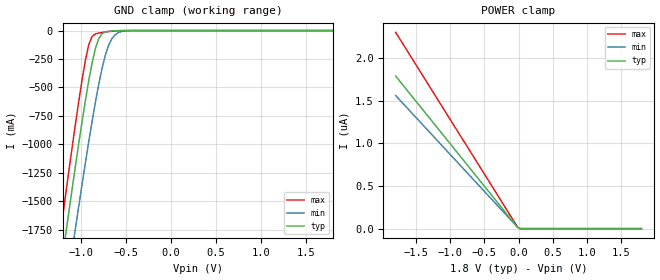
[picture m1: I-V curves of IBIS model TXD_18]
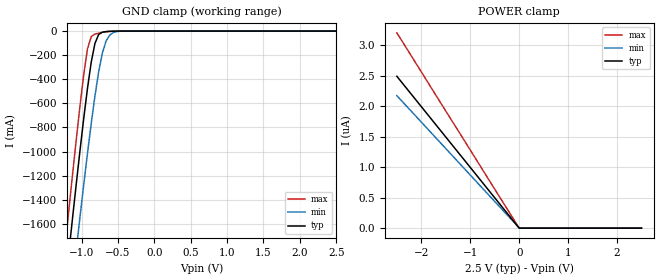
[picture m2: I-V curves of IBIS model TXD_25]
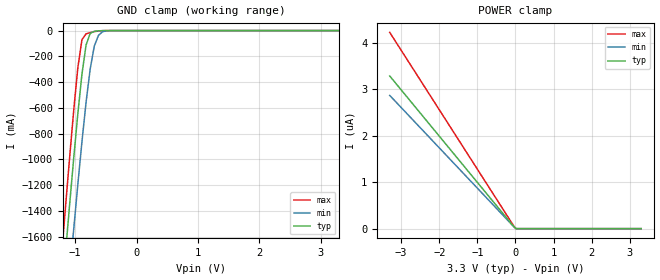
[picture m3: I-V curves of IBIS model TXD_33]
| IBIS file created by Layout Workbench Version 22.1.4.12161.401368   004
| Cadence Design Systems, Inc. 2011
[IBIS ver]   4.2
[File name]  iso6041.ibs
[File Rev]   1.5
[Date]   07 23, 2025
[Source]   Model built from TISPICED simulations at:
   Texas Instruments Incorporated.
   Analog-eLab, HPA 12500 TI Blvd
   Dallas, TX -75243
   For Support e-mail: elab_ibis@list.ti.com
[Notes]   This product is designed as an aid for customers of Texas Instruments.
   No warranties, either expressed or implied, with respect to this third party software (if any)
   or with respect to its fitness for any particular purpose is claimed by Texas Instruments or
   the author. The software (if any) is provided solely on an "as is" basis. The entire risk as to
   its quality and performance is with the customer
[Disclaimer]  This product is designed as an aid for customers of Texas Instruments. No warranties, either expressed or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
[Copyright] (C)Copyright 2025 Texas Instruments Incorporated. All rights reserved.
|   Component ISO60XX
[Component] ISO6041DW
[Manufacturer] Texas Instruments Incorporated
[Package]   |16-pin SOIC DW package
|   typ   min   max
R_pkg   0.04817   0.03432   0.09530
L_pkg   2.4595nH   1.6904nH   4.7034nH
C_pkg   0.847pF   0.428pF   1.397pF
[Pin]  signal_name   model_name   R_pin   L_pin   C_pin
1   VCC1   POWER   0.03455  3.39778n  0.89677p
2   GND1   GND   0.03432  3.12613n  0.84706p
3   INA   TXD1   0.04265  1.85523n  0.57831p
4   INB   TXD1   0.03948  1.69049n  0.59300p
5   INC   TXD1   0.03943  1.70546n  0.55709p
6   OUTD   RXD1   0.04257  1.86953n  0.56379p
7   EN1   TXDM1   0.04783  1.99000n  0.60148p
8   GND1   GND   0.03740  4.70338n  1.39696p
9   GND2   GND   0.03763  4.61305n  1.39587p
10   EN2   TXDM1   0.04703  2.01514n  0.58483p
11   IND   TXD2   0.07132  2.45946n  0.43321p
12   OUTC   RXD2   0.06147  2.13194n  0.42769p
13   OUTB   RXD2   0.07288  2.39260n  0.48001p
14   OUTA   RXD2   0.09530  3.03704n  0.47622p
15   GND2   GND   0.04817  4.23145n  0.93567p
16   VCC2   POWER   0.04790  4.51154n  0.99405p
[Model Selector] TXD1
TXD_18   TXD Input model for 1.71V - 1.89V
TXD_25   TXD Input model for 2.25V - 2.75V
TXD_33   TXD Input model for 3.0V - 3.6V
TXD_5   TXD Input model for 4.5V - 5.5V
[Model Selector] RXD1
RXD_18   RXD Output model for 1.71V - 1.89V
RXD_25   RXD Output model for 2.25V - 2.75V
RXD_33   RXD Output model for 3.0V - 3.6V
RXD_5   RXD Output model for 4.5V - 5.5V
[Model Selector] TXDM1
TXDM_18   TXD Input model for 1.71V - 1.89V
TXDM_25   TXD Input model for 2.25V - 2.75V
TXDM_33   TXD Input model for 3.15V - 3.6V
TXDM_5   TXD Input model for 4.5V - 5.5V
[Model Selector] TXD2
TXD_18   TXD Input model for 1.71V - 1.89V
TXD_25   TXD Input model for 2.25V - 2.75V
TXD_33   TXD Input model for 3.0V - 3.6V
TXD_5   TXD Input model for 4.5V - 5.5V
[Model Selector] RXD2
RXD_18   RXD Output model for 1.71V - 1.89V
RXD_25   RXD Output model for 2.25V - 2.75V
RXD_33   RXD Output model for 3.0V - 3.6V
RXD_5   RXD Output model for 4.5V - 5.5V
| Models and submodels in the file (12): TXD_18 (Input), TXD_25 (Input), TXD_33 (Input), TXD_5 (Input), TXDM_18 (Input), TXDM_25 (Input), TXDM_33 (Input), TXDM_5 (Input), RXD_18 (3-state), RXD_25 (3-state), RXD_33 (3-state), RXD_5 (3-state)
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|   TXD_18 Model
[Model]   TXD_18
Model_type   Input
|Signals   TXD
Vinl =  0.540V
Vinh =  1.260V
|   typ   min   max
C_comp   1.3pF   1.1pF   1.5pF
|   typ   min   max
[Temperature Range]   27   -55   150
[Voltage range]   1.8V   1.71V   1.89V
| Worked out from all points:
|   GND clamp passes 1 mA (typ) near -0.58 V on its own axis
[GND_clamp]
|Voltage   I(typ)   I(min)   I(max)
-1.8V     -5.506A    -5.93A     -5.269A
-1.245V   -2.234A    -2.756A    -1.895A
-1.208V   -2.022A    -2.55A     -1.676A
-1.171V   -1.811A    -2.345A    -1.459A
-1.06V    -1.194A    -1.742A    -825mA
-986mV    -801.2mA   -1.352A    -434mA
-912mV    -441.2mA   -978.2mA   -124.7mA
-838mV    -157.5mA   -630.6mA   -29.51mA
-764mV    -27.09mA   -331.9mA   -16.92mA
-690mV    -5.983mA   -125.6mA   -8.447mA
-542mV    -399.5uA   -6.689mA   -494.2uA
1.8V      0A         0A         -115nA
[POWER_clamp]
|Voltage   I(typ)   I(min)   I(max)
-1.8V     1.789uA    1.56uA     2.301uA
-13mV     12.95nA    15nA       16.65nA
24mV      0A         0A         0A
1.8V      0A         0A         0A
|   TXD_25 Model
[Model]   TXD_25
Model_type   Input
|Signals   TXD
Vinl =  0.750V
Vinh =  1.750V
|   typ   min   max
C_comp   1.3pF   1.1pF   1.5pF
|   typ   min   max
[Temperature Range]   27   -55   150
[Voltage range]   2.5V   2.25V   2.75V
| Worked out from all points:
|   GND clamp passes 1 mA (typ) near -0.58 V on its own axis
[GND_clamp]
|Voltage   I(typ)   I(min)   I(max)
-2.5V     -9.287A    -9.122A    -9.461A
-1.225V   -2.119A    -2.645A    -1.776A
-1.174V   -1.828A    -2.362A    -1.476A
-1.123V   -1.541A    -2.083A    -1.181A
-1.072V   -1.259A    -1.806A    -891.7mA
-1.021V   -984.1mA   -1.535A    -613.8mA
-919mV    -473.2mA   -1.013A    -146.1mA
-817mV    -102.7mA   -539.5mA   -24.7mA
-715mV    -9.204mA   -182mA     -10.99mA
-664mV    -3.989mA   -82.28mA   -6.169mA
-562mV    -642.2uA   -10.9mA    -884.6uA
2.5V      0A         0A         -319.8nA
[POWER_clamp]
|Voltage   I(typ)   I(min)   I(max)
-2.5V     2.488uA    2.171uA    3.199uA
1mV       0A         2.987nA    0A
52mV      0A         0A         0A
2.5V      0A         0A         0A
|   TXD_33 Model
[Model]   TXD_33
Model_type   Input
|Signals   TXD
Vinl =  0.990V
Vinh =  2.310V
|   typ   min   max
C_comp   1.3pF   1.1pF   1.5pF
|   typ   min   max
[Temperature Range]   27   -55   150
[Voltage range]   3.3V   3.0V   3.6V
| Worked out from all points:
|   GND clamp passes 1 mA (typ) near -0.57 V on its own axis
[GND_clamp]
|Voltage   I(typ)   I(min)   I(max)
-3.3V     -12.37A    -12.1A     -12.66A
-1.223V   -2.107A    -2.633A    -1.764A
-1.156V   -1.727A    -2.263A    -1.371A
-1.089V   -1.353A    -1.898A    -987mA
-1.022V   -989.5mA   -1.54A     -619.1mA
-955mV    -645mA     -1.193A    -287.8mA
-888mV    -337.4mA   -861.8mA   -70.28mA
-821mV    -112mA     -556.5mA   -25.45mA
-754mV    -21.16mA   -297.6mA   -15.62mA
-687mV    -5.702mA   -119.8mA   -8.165mA
-553mV    -522.6uA   -8.764mA   -688.5uA
3.3V      0A         0A         -383.9nA
[POWER_clamp]
|Voltage   I(typ)   I(min)   I(max)
-3.3V     3.286uA    2.868uA    4.224uA
-50mV     49.84nA    47.39nA    64.06nA
17mV      0A         0A         0A
3.3V      0A         0A         0A
